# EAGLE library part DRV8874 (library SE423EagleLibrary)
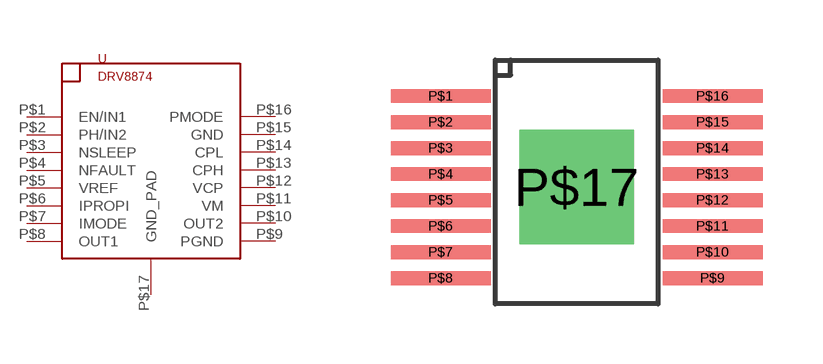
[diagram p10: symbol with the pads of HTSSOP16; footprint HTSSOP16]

Designator prefix U

## DRV8874  [HTSSOP16]
P$1  EN/IN1
P$2  PH/IN2
P$3  NSLEEP
P$4  NFAULT
P$5  VREF
P$6  IPROPI
P$7  IMODE
P$8  OUT1
P$9  PGND
P$10  OUT2
P$11  VM
P$12  VCP
P$13  CPH
P$14  CPL
P$15  GND
P$16  PMODE
P$17  GND_PAD

## Footprint HTSSOP16 (pad centres in mm)
smd 2.5 x 0.35: P$1 -3.4,2.275; P$2 -3.4,1.625; P$3 -3.4,0.975; P$4 -3.4,0.325; P$5 -3.4,-0.325; P$6 -3.4,-0.975; P$7 -3.4,-1.625; P$8 -3.4,-2.275; P$9 3.4,-2.275; P$10 3.4,-1.625; P$11 3.4,-0.975; P$12 3.4,-0.325; P$13 3.4,0.325; P$14 3.4,0.975; P$15 3.4,1.625; P$16 3.4,2.275
drill 1.905 pad 2.54 square: P$17 0,0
